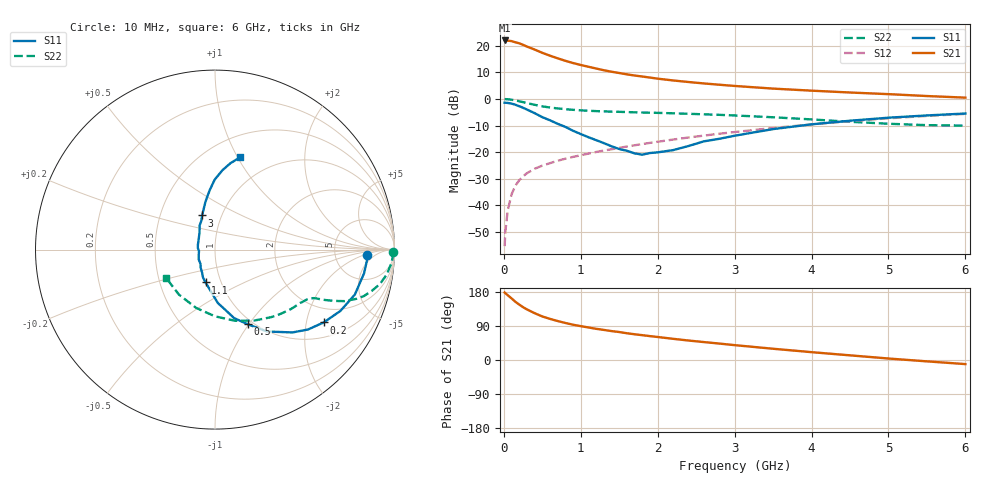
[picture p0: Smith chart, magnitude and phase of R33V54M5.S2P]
! SIEMENS Small Signal Semiconductors
! BFR181
! Si NPN RF Bipolar Junction Transistor in SOT23
! VCE = 3.5 V  IC = 4.5 mA
! Common Emitter S-Parameters:  May  1996
# GHz  S  MA  R  50
!  f  S11  S21  S12  S22
! GHz  MAG  ANG  MAG  ANG  MAG  ANG  MAG  ANG
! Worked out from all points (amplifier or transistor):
!   36 points, 10 MHz to 6 GHz, reference 50 ohm
!   highest |S21| = 22.0 dB at 10 MHz (marker M1)
!   |S21| within 3 dB of that: start of sweep to 362.9 MHz
!   unconditionally stable (mu >= 1): 1.187 GHz to 3.021 GHz
!   at 250 MHz: K = 0.39, MSG = 24.7 dB, |S12| = -29.1 dB
!   at 1.4 GHz: K = 1.04, MAG = 13.3 dB, |S12| = -18.9 dB
!   at 6 GHz: K = 0.86, MSG = 3.1 dB, |S12| = -5.6 dB
!   S11 on the Smith chart (normalised r, x): 10 MHz: 12, -2; 200 MHz: 1.46, -2.54; 500 MHz: 0.94, -0.99; 1.1 GHz: 0.84, -0.32; 3 GHz: 0.81, +0.32; 6 GHz: 0.71, +1.02
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0.01  0.8494 -1.9  12.59 178.0  0.0017 92.2  0.9935 -0.8
0.02  0.8501 -3.5  12.39 176.1  0.0032 87.8  0.9922 -1.8
0.05  0.841 -9.0  12.5 171.0  0.0079 86.2  0.9868 -4.2
0.1  0.8186 -17.8  12.24 162.6  0.016 82.6  0.9674 -8.2
0.15  0.7776 -26.1  11.63 153.6  0.0234 75.4  0.9388 -11.8
0.2  0.7291 -33.8  11.13 146.2  0.0295 72.9  0.9039 -14.7
0.25  0.6829 -40.7  10.41 139.4  0.035 69.5  0.8694 -17.3
0.3  0.632 -46.9  9.672 133.5  0.0401 68.2  0.8364 -19.1
0.4  0.5405 -57.6  8.495 123.6  0.0485 64.8  0.7766 -21.7
0.5  0.4541 -66.3  7.369 114.9  0.0557 63.4  0.7259 -23.2
0.6  0.3964 -74.4  6.508 108.5  0.0619 62.4  0.689 -24.2
0.8  0.2984 -86.9  5.214 97.7  0.0751 61.8  0.6414 -25.4
0.9  0.2522 -92.7  4.735 93.1  0.0813 62.3  0.6243 -25.8
1.1  0.1904 -106.1  4.029 85.8  0.0937 63.1  0.5997 -27.0
1.3  0.1475 -119.1  3.467 79.4  0.107 63.2  0.5831 -28.4
1.6  0.1058 -148.9  2.9 70.6  0.1273 63.3  0.5665 -31.1
2.2  0.1089 146.2  2.227 55.9  0.1721 62.1  0.5371 -38.1
3  0.2031 110.7  1.755 39.2  0.2383 57.9  0.4889 -50.4
3.5  0.2709 101.4  1.564 29.7  0.284 54.1  0.4522 -60.9
4.5  0.3894 90.3  1.321 12.3  0.3821 44.0  0.3717 -90.0
5.5  0.4895 79.8  1.134 -3.6  0.4791 31.4  0.3212 -128.7
6  0.5318 74.9  1.058 -10.8  0.5232 24.3  0.3151 -150.0
